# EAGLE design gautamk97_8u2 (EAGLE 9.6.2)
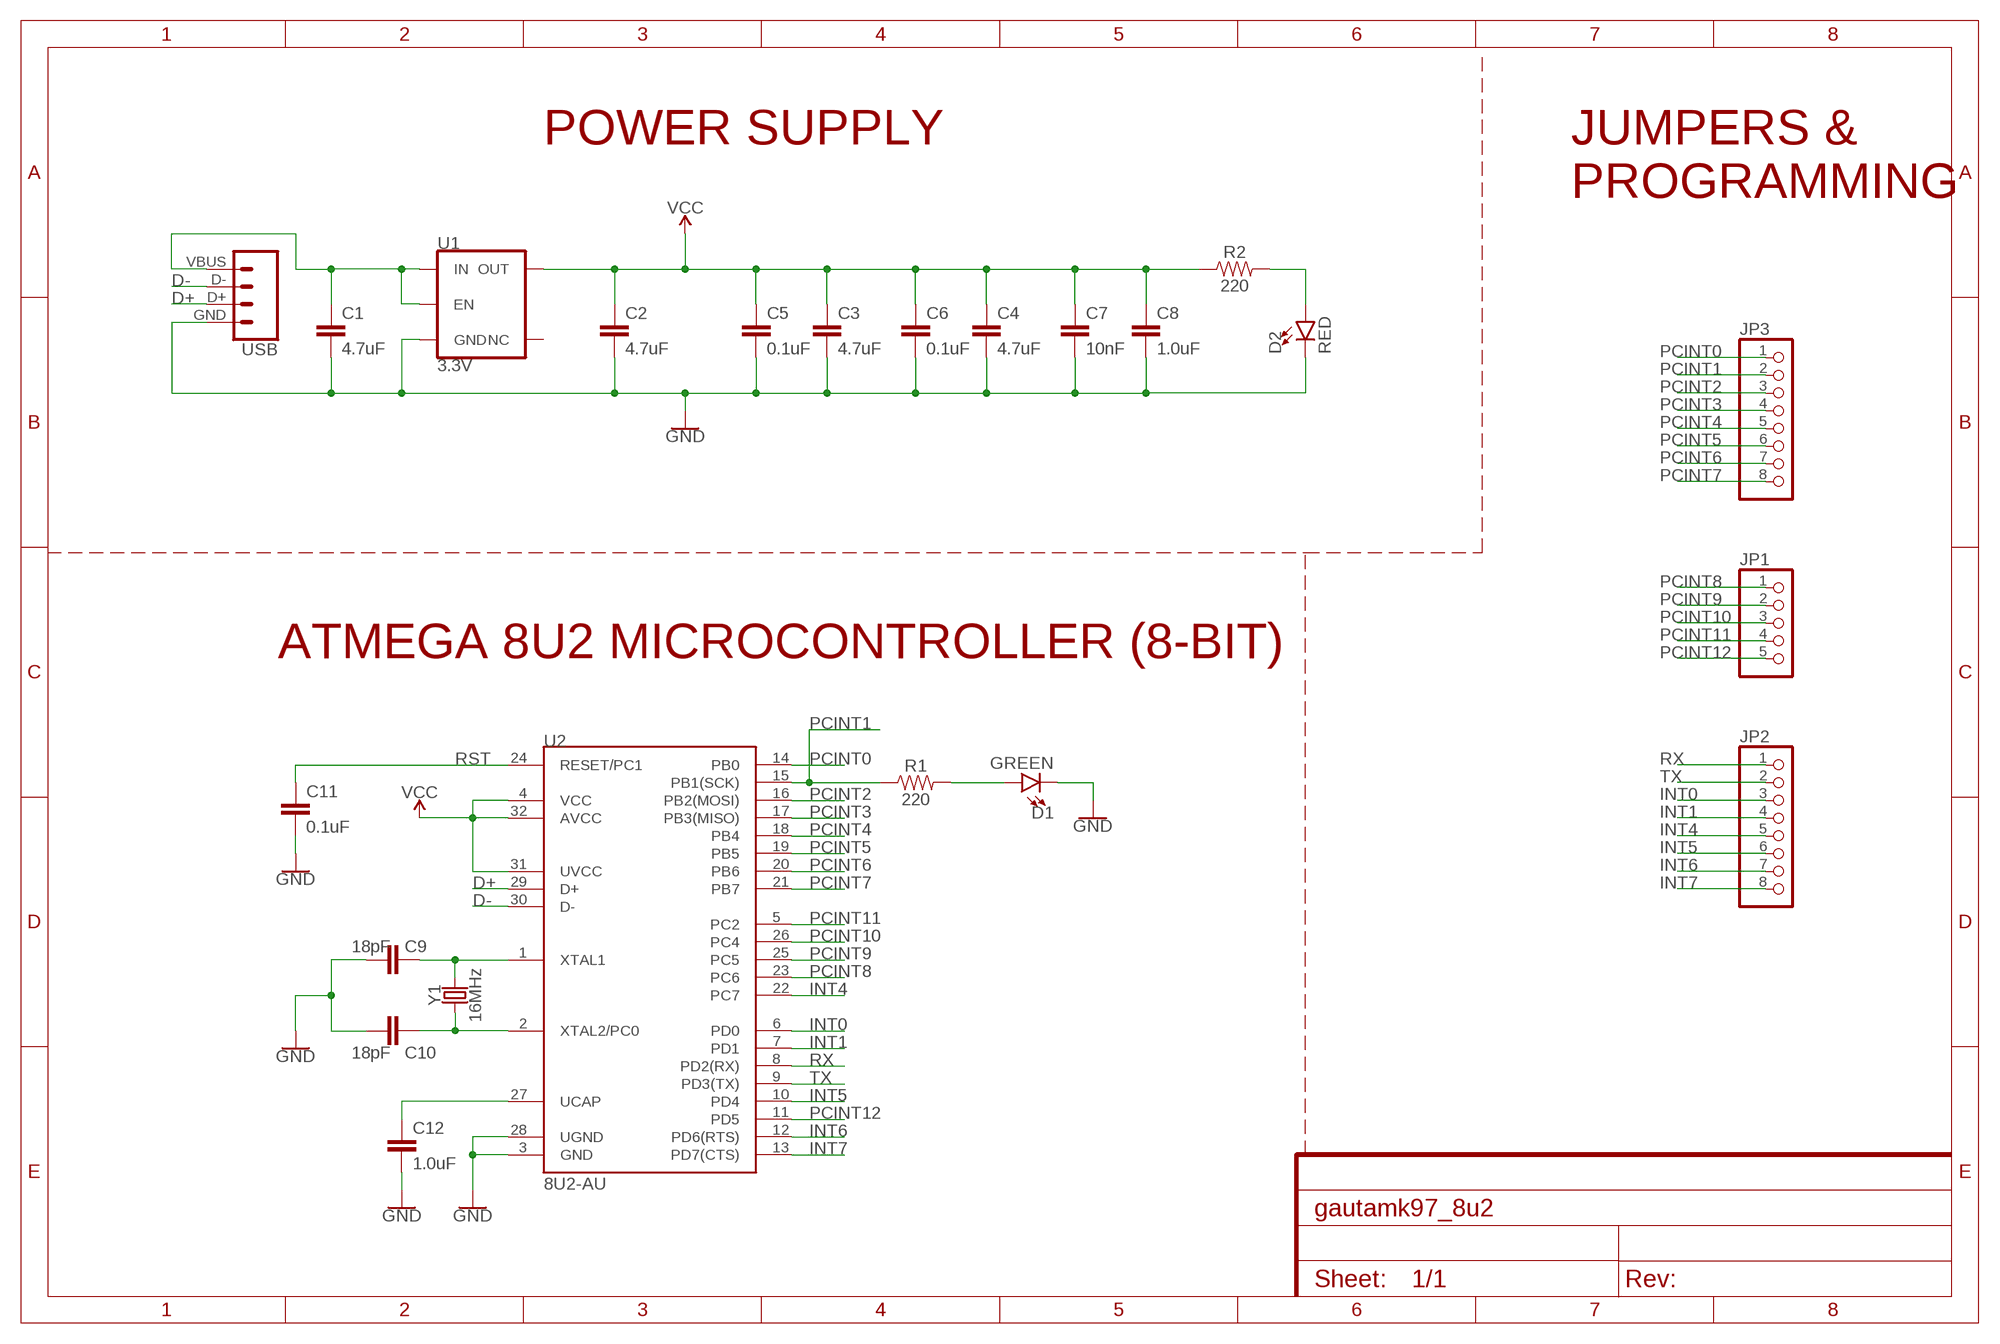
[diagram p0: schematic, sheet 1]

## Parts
C1  4.7uF  4.7UF-0603-6.3V-(10%)  [0603]
C2  4.7uF  4.7UF-0603-6.3V-(10%)  [0603]
C3  4.7uF  4.7UF-0603-6.3V-(10%)  [0603]
C4  4.7uF  4.7UF-0603-6.3V-(10%)  [0603]
C5  0.1uF  0.1UF-0603-25V-5%  [0603]
C6  0.1uF  0.1UF-0603-25V-5%  [0603]
C7  10nF  10NF-0603-50V-10%  [0603]
C8  1.0uF  1.0UF-0603-16V-10%  [0603]
C9  18pF  18PF-0603-50V-5%  [0603]
C10  18pF  18PF-0603-50V-5%  [0603]
C11  0.1uF  0.1UF-0603-25V-5%  [0603]
C12  1.0uF  1.0UF-0603-16V-10%  [0603]
D1  GREEN  LED-GREEN0603  [LED-0603]
D2  RED  LED-RED0603  [LED-0603]
JP1  PINHD-1X5  [1X05]
JP2  PINHD-1X8  [1X08]
JP3  PINHD-1X8  [1X08]
R1  220  220OHM-0603-1/10W-1%  [0603]
R2  220  220OHM-0603-1/10W-1%  [0603]
U1  3.3V  V_REG_AP2112K-3.3V  [SOT23-5]
U2  8U2-AU  ATMEGA8U2AU  [TQFP32-08_MCU]
USB  USB_SOLDER_PADS  [USB-SOLDER-PADS]
Y1  16MHz  CRYSTAL-16MHZSMD-2X1.6  [CRYSTAL-SMD-2.0X1.6MM]

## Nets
D+: U2.29(D+) USB.D+
D-: U2.30(D-) USB.D-
GND: C1.2 C2.2 C3.2 C4.2 C5.2 C6.2 C7.2 C8.2 C9.2 C10.2 C11.2 C12.2 D1.C D2.C U1.2(GND) U2.3(GND) U2.28(UGND) USB.GND
INT0: JP2.3 U2.6(PD0)
INT1: JP2.4 U2.7(PD1)
INT4: JP2.5 U2.22(PC7)
INT5: JP2.6 U2.10(PD4)
INT6: JP2.7 U2.12(PD6(RTS))
INT7: JP2.8 U2.13(PD7(CTS))
N$2: C1.1 U1.1(IN) U1.3(EN) USB.VBUS
N$3: C12.1 U2.27(UCAP)
N$4: D1.A R1.2
N$5: D2.A R2.2
N$7: C9.1 U2.1(XTAL1) Y1.3
N$8: C10.1 U2.2(XTAL2/PC0) Y1.1
PCINT0: JP3.1 U2.14(PB0)
PCINT1: JP3.2 R1.1 U2.15(PB1(SCK))
PCINT2: JP3.3 U2.16(PB2(MOSI))
PCINT3: JP3.4 U2.17(PB3(MISO))
PCINT4: JP3.5 U2.18(PB4)
PCINT5: JP3.6 U2.19(PB5)
PCINT6: JP3.7 U2.20(PB6)
PCINT7: JP3.8 U2.21(PB7)
PCINT8: JP1.1 U2.23(PC6)
PCINT9: JP1.2 U2.25(PC5)
PCINT10: JP1.3 U2.26(PC4)
PCINT11: JP1.4 U2.5(PC2)
PCINT12: JP1.5 U2.11(PD5)
RST: C11.1 U2.24(RESET/PC1)
RX: JP2.1 U2.8(PD2(RX))
TX: JP2.2 U2.9(PD3(TX))
VCC: C2.1 C3.1 C4.1 C5.1 C6.1 C7.1 C8.1 R2.1 U1.5(OUT) U2.4(VCC) U2.31(UVCC) U2.32(AVCC)
Unconnected: U1.4(NC)

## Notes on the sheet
- POWER SUPPLY
- JUMPERS &
  PROGRAMMING
- ATMEGA 8U2 MICROCONTROLLER (8-BIT)

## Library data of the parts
C1-C4 = SparkFun-Capacitors:4.7UF: 4.7µF ceramic capacitors; PROD_ID: CAP-08280
C5 C6 C11 = SparkFun-Capacitors:0.1UF: 0.1µF ceramic capacitors; PROD_ID: CAP-08604
C7 = SparkFun-Capacitors:10NF: 0.01uF/10nF/10,000pF ceramic capacitors; PROD_ID: CAP-00867
C8 C12 = SparkFun-Capacitors:1.0UF: 1µF ceramic capacitors; PROD_ID: CAP-00868
C9 C10 = SparkFun-Capacitors:18PF: 18pF ceramic capacitors; PROD_ID: CAP-08267
D1 = SparkFun-LED:LED-GREEN: Green SMD LED; PROD_ID: DIO-00821
D2 = SparkFun-LED:LED-RED: Red SMD LED; PROD_ID: DIO-00819
JP1 = pinhead:PINHD-1X5: PIN HEADER
JP2 JP3 = pinhead:PINHD-1X8: PIN HEADER
R1 R2 = SparkFun-Resistors:220OHM: 220Ω resistor; PROD_ID: RES-07861
U1 = SparkFun-IC-Power:V_REG_AP2112: AP2112 - 600mA CMOS LDO Regulator w/ Enable The AP2112 is CMOS process low dropout linear regulator with enable function, the regulator delivers a guaranteed 600mA (min.) continuous load current. Features Output Voltage Accuracy: ±1.5% Output Current: 600mA (Min.) Foldback Short Current Protection: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; PROD_ID: VREG-12457
U2 = SparkFun-Retired:ATMEGA8U2: Atmel 32-pin 8-bit Microcontroller with 8/16/32K Bystes of ISP Flash and USB Controller. ATmega8U2, ATmega16U2, and ATmega32U2 Datasheet SparkFun Products Storefront component: ATMEGA8U2-AU (COM-13703); PROD_ID: IC-10104
USB = SparkFun-Connectors:USB_SOLDER_PADS: Solder pad access to USB pins. Helpful to expose on PCBs so user can attach external USB connector if necessary.
Y1 = SparkFun-Clocks:CRYSTAL-16MHZ: 16MHz Crystal; PROD_ID: XTAL-14681

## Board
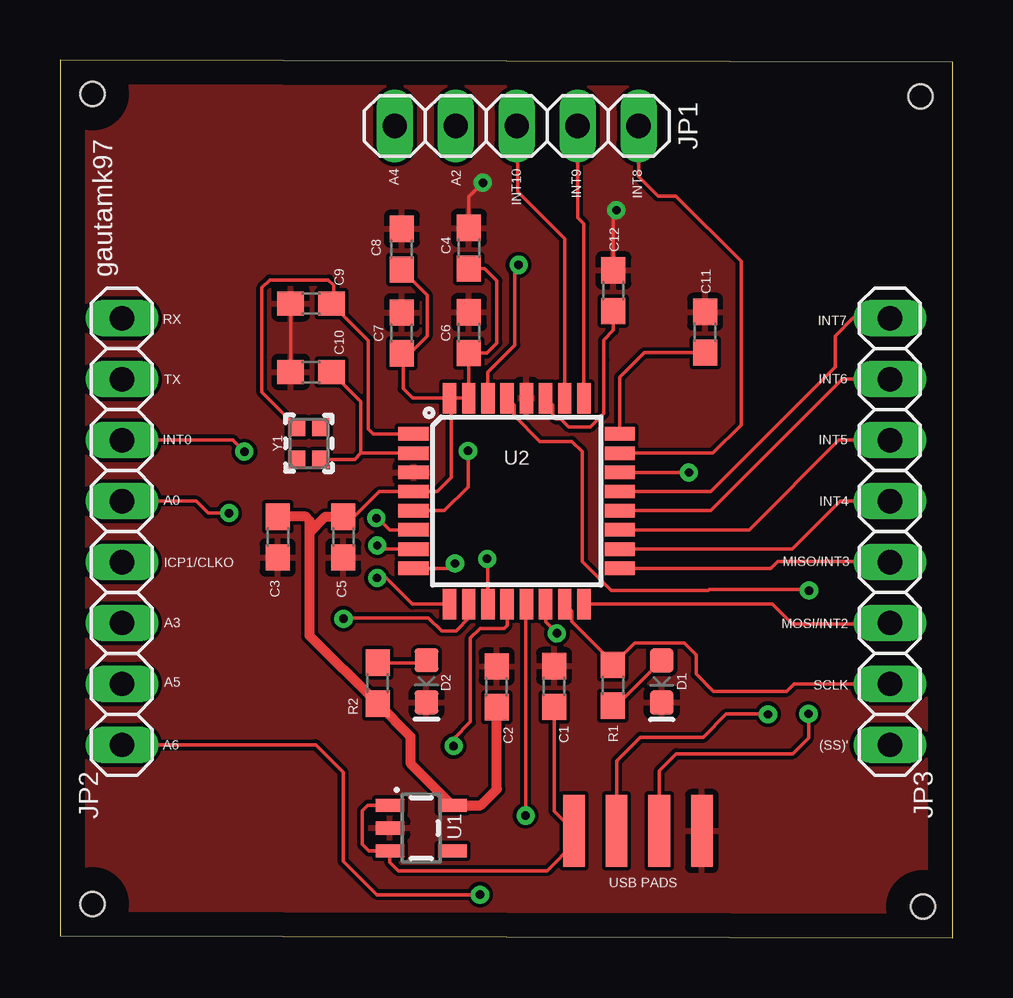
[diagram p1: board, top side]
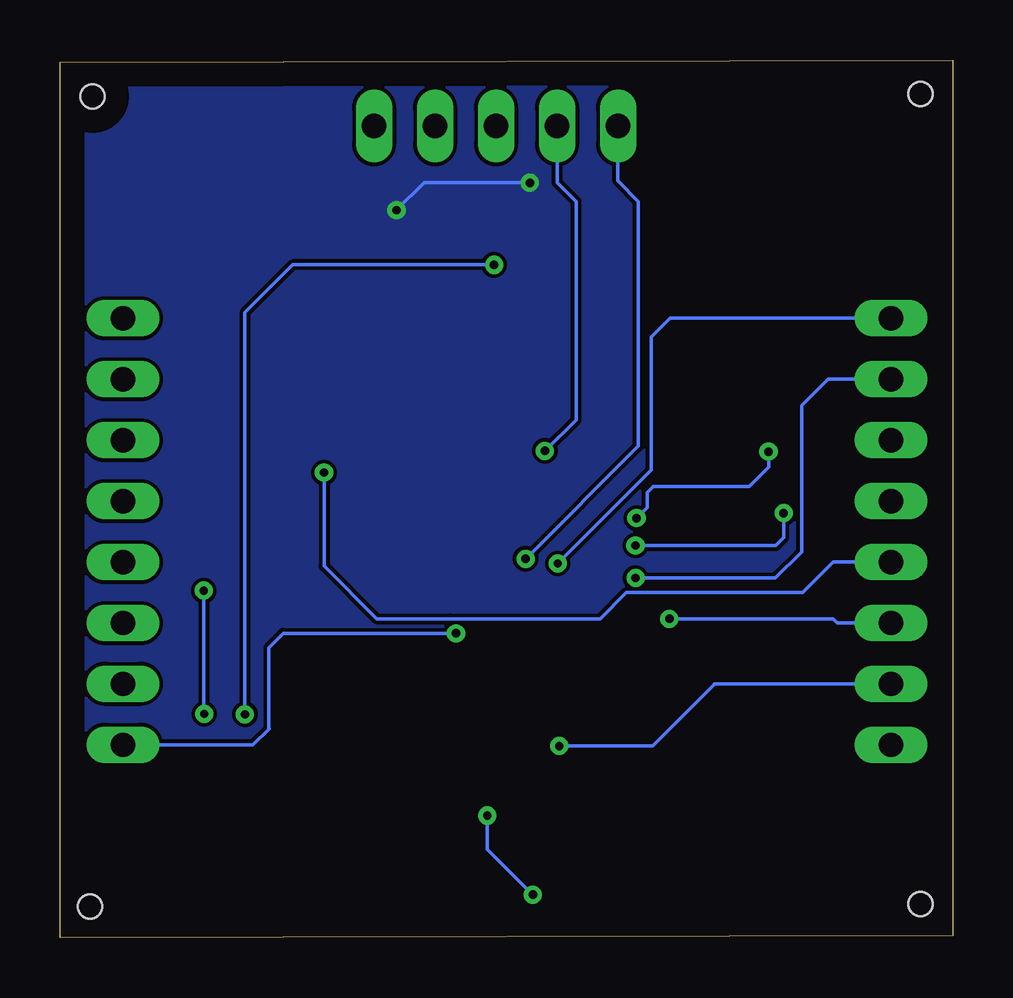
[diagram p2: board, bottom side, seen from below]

Size 37.2 x 36.6 mm. Coordinates in mm from the lower left corner, seen from the top.
Outline: 0,0.1 37.2,0 37.2,36.5 0,36.6 0,0.1
Copper layers (1*16): Top 0.035mm / dielectric 1.5mm / Bottom 0.035mm
Design rules "default": minimum track width 6mil, minimum drill 0.35mm, track to track 6mil, track to pad 6mil, pad to pad 6mil, via to via 6mil, smd to smd 6mil, copper to edge 40mil, drill to drill 6mil, minimum pad ring 10mil, minimum via ring 8mil, stop-mask expansion 4mil, vias tented up to drill 0mil, thermal gap 10mil
Holes 1 mm at 35.85,35.08 1.35,35.18 1.35,1.42 35.95,1.31

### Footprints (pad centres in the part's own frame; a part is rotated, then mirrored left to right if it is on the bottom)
0603 = smd 1.1 x 1: 1 -0.85,0; 2 0.85,0
LED-0603 = smd 1 x 1: A -0.877,0; C 0.877,0
1X05 = drill 1.016 long: 1 -5.08,0; 2 -2.54,0; 3 0,0; 4 2.54,0; 5 5.08,0
1X08 = drill 1.016 long: 1 -8.89,0; 2 -6.35,0; 3 -3.81,0; 4 -1.27,0; 5 1.27,0; 6 3.81,0; 7 6.35,0; 8 8.89,0
SOT23-5 = smd 0.55 x 1.2: 1 -0.95,-1.3; 2 0,-1.3; 3 0.95,-1.3; 4 0.95,1.3; 5 -0.95,1.3
TQFP32-08_MCU = smd 1.27 x 0.559: 1 -4.293,2.8; 2 -4.293,2; 3 -4.293,1.2; 4 -4.293,0.4; 5 -4.293,-0.4; 6 -4.293,-1.2; 7 -4.293,-2; 8 -4.293,-2.8; 17 4.293,-2.8; 18 4.293,-2; 19 4.293,-1.2; 20 4.293,-0.4; 21 4.293,0.4; 22 4.293,1.2; 23 4.293,2; 24 4.293,2.8 | smd 0.559 x 1.27: 9 -2.8,-4.293; 10 -2,-4.293; 11 -1.2,-4.293; 12 -0.4,-4.293; 13 0.4,-4.293; 14 1.2,-4.293; 15 2,-4.293; 16 2.8,-4.293; 25 2.8,4.293; 26 2,4.293; 27 1.2,4.293; 28 0.4,4.293; 29 -0.4,4.293; 30 -1.2,4.293; 31 -2,4.293; 32 -2.8,4.293
USB-SOLDER-PADS = smd 3 x 0.9: D+ 0,-0.889; D- 0,0.889; GND 0,-2.667; VBUS 0,2.667
CRYSTAL-SMD-2.0X1.6MM = smd 0.75 x 0.7: 1 -0.675,-0.5; 2 0.675,-0.5; 3 0.675,0.5; 4 -0.675,0.5

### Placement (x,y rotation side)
C1  20.59,10.48 90 top
C2  18.19,10.47 90 top
C3  9.07,16.71 270 top
C4  17.04,28.75 90 top
C5  11.81,16.71 270 top
C6  17.04,25.23 90 top
C7  14.24,25.22 90 top
C8  14.24,28.71 90 top
C9  10.46,26.45 180 top
C10  10.46,23.59 180 top
C11  26.88,25.25 90 top
C12  23.06,26.98 90 top
D1  25.07,10.69 270 top
D2  15.27,10.7 270 top
JP1  19.03,33.85 180 top
JP2  2.58,16.94 270 top
JP3  34.58,16.94 90 top
R1  23.03,10.53 270 top
R2  13.23,10.62 90 top
U1  15.05,4.58 270 top
U2  19.03,18.21 0 top
USB  24.08,4.46 90 top
Y1  10.37,20.62 90 top

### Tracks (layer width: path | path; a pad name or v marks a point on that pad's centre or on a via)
D+  (via drill 0.35)
  Top 0.152: U2.29 18.92,22.21 18.92,21.77 19.99,20.7 21.32,20.7 21.75,20.27 21.75,15.69 22.96,14.48 27.02,14.48 27.06,14.52 31.17,14.52 v31.21,14.48 | USB.D+ 24.97,6.97 25.68,7.68 30.53,7.68 31.19,8.34 v31.19,9.34
  Bottom 0.152: v31.21,14.48 31.21,9.34 v31.19,9.34
D-  (via drill 0.35)
  Top 0.152: U2.30 17.83,23.6 18.95,24.72 18.95,27.96 19.08,28.09 v19.11,28.06 | USB.D- 23.19,7.38 24.18,8.37 26.81,8.37 27.77,9.33 v29.51,9.33 29.52,9.32 v29.5,9.32
  Bottom 0.152: v19.11,28.06 27.5,28.06 29.5,26.06 v29.5,9.32
GND  (via drill 0.35)
  Top 0.152: C12.2 23.06,30.42 23.08,30.44 v23.18,30.34 | v17.62,31.48 17.04,30.9 C4.2 | C9.2 C10.2
  Bottom 0.152: v23.18,30.34 22.03,31.49 v17.62,31.49 v17.62,31.48
  pour Bottom: 0,36.6 0,0 37.3,0 37.3,36.5 37.4,36.6 0.1,36.6
  pour Top: 0,36.7 0,0.1 0.1,0 37.3,0 37.3,36.6 0.2,36.6 0.1,36.5
INT0  (via drill 0.35)
  Top 0.152: U2.6 13.73,17.01 13.24,17.5 v13.18,17.5 | v7.68,20.27 7.22,20.73 7.22,20.75 JP2.3
  Bottom 0.152: v13.18,17.5 12.74,17.94 12.74,18.56 12.49,18.81 8.49,18.81 7.67,19.63 v7.67,20.27 v7.68,20.27
INT1  (via drill 0.35)
  Top 0.152: U2.7 13.41,16.21 13.24,16.38 v13.22,16.36 | v7.05,17.71 6.17,17.71 5.67,18.21 JP2.4
  Bottom 0.152: v13.22,16.36 7.38,16.36 7.05,16.69 v7.05,17.71
INT4  (via drill 0.35)
  Top 0.152: U2.22 v26.19,19.41 v26.2,19.4
  Bottom 0.152: v26.2,19.4 26.2,15.5 24,13.3 20.96,13.3 20.95,13.31 14.69,13.31 13.6,14.4 6.26,14.4 4.99,15.67 JP2.5
INT5  (via drill 0.35)
  Top 0.152: U2.10 17.03,13.33 16.5,12.8 15.9,12.8 15.35,13.35 11.88,13.35 11.83,13.3 v11.81,13.3
  Bottom 0.152: JP2.6 4.81,13.13 4.98,13.3 v11.81,13.3
INT6  (via drill 0.35)
  Top 0.152: v16.4,8 16.4,8.3 17.1,9 17.1,12.5 17.5,12.9 18.5,12.9 18.63,13.03 U2.12
  Bottom 0.152: v16.4,8 12.5,8 9.93,10.57 9.93,10.59 JP2.7
INT7  (via drill 0.35)
  Top 0.152: JP2.8 10.65,8.05 11.8,6.9 11.8,3.2 13.2,1.8 v17.5,1.8 | v19.4,5.1 19.4,13.89 U2.13
  Bottom 0.152: v17.5,1.8 19.4,3.7 v19.4,5.1
N$2
  Top 0.152: C1.1 20.59,5.28 USB.VBUS 21.41,3.91 20.3,2.8 14.1,2.8 13.75,3.15 U1.3 12.87,3.63 12.6,3.9 12.6,5.3 12.83,5.53 U1.1
N$3
  Top 0.152: C12.1 23.06,25.33 22.65,24.92 22.65,24.1 22.66,24.09 22.66,21.87 22.09,21.3 21.2,21.3 20.86,21.64 20.66,21.64 20.52,21.77 20.52,22.21 U2.27
N$4
  Top 0.152: R1.2 23.18,9.68 D1.A
N$5
  Top 0.152: D2.A 15.16,11.47 R2.2
N$7
  Top 0.152: Y1.3 8.41,22.75 8.41,27.11 8.73,27.43 11.18,27.43 11.4,27.21 11.4,26.54 C9.1 12.85,24.91 12.85,21.21 13.05,21.01 U2.1
N$8
  Top 0.152: U2.2 12.54,20.21 | 12.54,20.21 12.53,20.22 12.53,22.37 C10.1 | 12.54,20.21 12.27,19.95 Y1.1
PCINT0  (via drill 0.35)
  Top 0.152: v20.7,12.7 20.23,13.17 U2.14
  Bottom 0.152: v20.7,12.7 27.9,12.7 28.5,12.1 28.5,8.72 28.49,8.71 29.16,8.04 JP3.1
PCINT1
  Top 0.152: JP3.2 30.59,10.59 30.28,10.28 27.22,10.28 26.5,11 26.5,11.8 26,12.3 23.95,12.3 R1.1 23.03,11.48 21.32,13.19 21.32,13.63 U2.15
PCINT2
  Top 0.152: U2.16 29.68,13.92 30.5,13.1 34.55,13.1 JP3.3
PCINT3
  Top 0.152: U2.17 29.61,15.41 29.9,15.7 34.55,15.7 JP3.4
PCINT4
  Top 0.152: U2.18 30.51,16.21 32.51,18.21 JP3.5
PCINT5
  Top 0.152: U2.19 28.71,17.01 32.45,20.75 JP3.6
PCINT6
  Top 0.152: U2.20 27.11,17.81 32.6,23.3 JP3.7
PCINT7
  Top 0.152: U2.21 27.11,18.61 32.3,23.8 32.3,25.1 33.03,25.83 JP3.8
PCINT8
  Top 0.152: U2.23 27.2,20.21 28.38,21.39 28.38,28.21 25.66,30.93 24.92,30.93 24.11,31.74 JP1.1
PCINT9
  Top 0.152: U2.25 21.83,29.77 21.57,30.03 JP1.2
PCINT10
  Top 0.152: U2.26 21.03,29.15 19.07,31.11 19.07,33.81 JP1.3
PCINT11  (via drill 0.35)
  Top 0.152: U2.5 16.01,17.81 17,18.8 v17,20.3
  Bottom 0.152: v17,20.3 15.7,21.6 15.7,30.7 16.49,31.49 JP1.4
PCINT12  (via drill 0.35)
  Top 0.152: U2.11 17.83,15.77 v17.8,15.8
  Bottom 0.152: v17.8,15.8 13.1,20.5 13.1,30.7 13.96,31.56 JP1.5
RST
  Top 0.152: U2.24 23.32,23.37 24.35,24.4 C11.1
RX  (via drill 0.35)
  Top 0.152: U2.8 16.25,15.41 v16.45,15.61 v16.46,15.61
  Bottom 0.152: v16.46,15.61 12.57,19.5 12.57,25.04 11.78,25.83 JP2.1
TX  (via drill 0.35)
  Top 0.152: U2.9 14.68,13.92 13.62,14.98 13.22,14.98 13.21,14.97 v13.21,15 v13.22,15.01
  Bottom 0.152: JP2.2 5.2,23.3 6.3,22.2 6.3,16.1 7.39,15.01 v13.22,15.01
VCC
  Top 0.152: C2.1 | 10.4,17.4 10.24,17.56 | C5.1 12.26,17.56 13.31,18.61 U2.4 15.71,18.61 16.3,19.2 16.3,22.43 U2.32 | C7.1 14.3,24.31 14.3,24.3 | 14.3,24.3 14.3,22.9 14.7,22.5 U2.32 | U2.32 U2.31 17.04,22.51 C6.1 17.78,24.38 18.2,24.8 18.2,27.4 17.7,27.9 C4.1 | C8.1 15.3,26.8 15.3,25.09 14.51,24.3 14.3,24.3
  Top 0.406: C2.1 18.2,6.2 17.53,5.53 U1.5 14.6,7.28 14.6,8.4 R2.1 10.4,12.6 10.4,16.9 | 10.24,17.56 C3.1 | 10.4,16.9 10.4,17.4 | C5.1 11.06,17.56 10.4,16.9

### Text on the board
tNames: gautamk97 | A4 | A2 | INT9 | INT8 | INT10 | INT7 | RX | TX | INT6 | INT5 | INT0 | A0 | INT4 | MISO/INT3 | ICP1/CLKO | A3 | MOSI/INT2 | A5 | SCLK | A6 | (SS)' | USB PADS

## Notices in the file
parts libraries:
SparkFun-Connectors: Licensing: Creative Commons ShareAlike 4.0 International - https://creativecommons.org/licenses/by-sa/4.0
